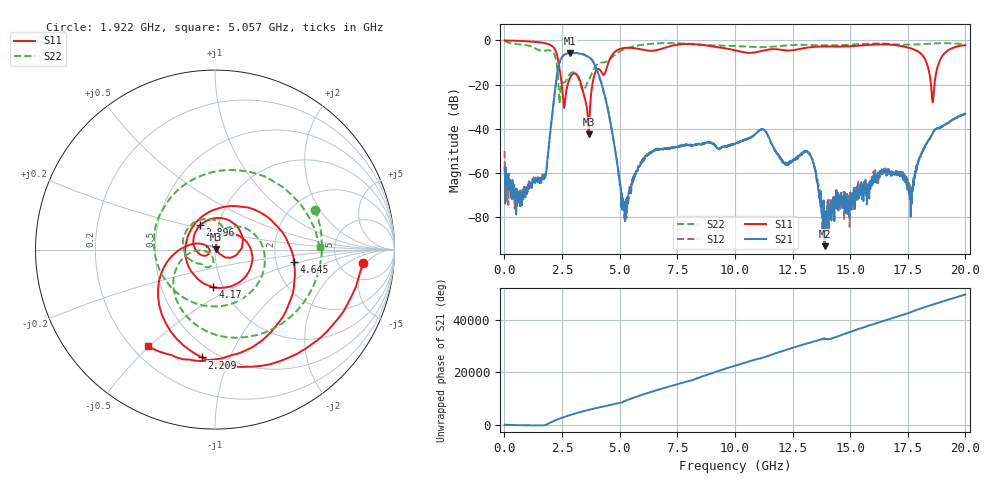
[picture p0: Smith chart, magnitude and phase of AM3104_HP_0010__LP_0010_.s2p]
!Created with skrf (http://scikit-rf.org).
# Hz S RI R 50.0
!freq ReS11 ImS11 ReS21 ImS21 ReS12 ImS12 ReS22 ImS22
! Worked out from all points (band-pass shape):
!   1601 points, 10 MHz to 20 GHz, reference 50 ohm
!   highest |S21| = -5.67 dB at 2.846 GHz (marker M1); lowest = -93.2 dB at 13.89 GHz (marker M2)
!   |S21| within 3 dB of the highest: 2.437 GHz to 3.787 GHz (1.35 GHz wide, 43.4 % of centre)
!   lowest |S11| = -42.5 dB at 3.658 GHz (marker M3), VSWR 1.02, Z = 50.7 + j0.166 ohm
!   |S11| at or under -10 dB: 2.351 GHz to 4.513 GHz (2.161 GHz wide, 63 % of centre); 18.31 GHz to 18.85 GHz (545.4 MHz wide, 2.94 % of centre)
!   |S22| runs from -28.6 to -0.2 dB; largest |S21 - S12| = 0.004
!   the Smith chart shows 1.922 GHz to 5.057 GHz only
!   S11 on the Smith chart (normalised r, x): 1.922 GHz: 8.63, -3.99; 2.209 GHz: 0.42, -0.79; 2.896 GHz: 0.82, +0.23; 4.17 GHz: 0.90, -0.39; 4.645 GHz: 2.52, -0.42; 5.057 GHz: 0.26, -0.50
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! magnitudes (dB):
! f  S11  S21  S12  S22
! 10 MHz  0.0  -57.8  -50.1  -0.2
! 647.2 MHz  -0.2  -68.6  -69.7  -1.8
! 1.922 GHz  -1.7  -48.6  -48.7  -4.4
! 2.209 GHz  -4.4  -21.5  -21.5  -7.5
! 2.584 GHz  -30.3  -6.6  -6.6  -19.1
! 2.846 GHz  -16.9  -5.7  -5.7  -15.2
! 2.896 GHz  -16.0  -5.7  -5.7  -14.7
! 3.346 GHz  -20.5  -6.1  -6.1  -21.4
! 3.658 GHz  -42.5  -7.5  -7.5  -18.1
! 4.17 GHz  -13.6  -18.0  -18.0  -10.0
! 4.645 GHz  -7.0  -39.6  -39.8  -7.9
! 5.057 GHz  -3.7  -69.2  -69.2  -4.7
! 5.245 GHz  -3.3  -73.2  -81.7  -3.8
! 6.682 GHz  -4.2  -49.4  -49.1  -1.3
! 10.01 GHz  -4.4  -46.9  -46.6  -2.5
! 13.34 GHz  -3.0  -53.3  -53.5  -2.1
! 13.89 GHz  -2.7  -93.2  -80.4  -2.2
! 16.68 GHz  -1.8  -60.4  -59.9  -1.5
! 17.64 GHz  -3.6  -75.5  -68.4  -1.9
! 18.59 GHz  -28.0  -41.9  -42.0  -1.4
! 19.03 GHz  -6.6  -38.8  -38.8  -1.2
! 20 GHz  -2.2  -33.2  -33.2  -1.7
